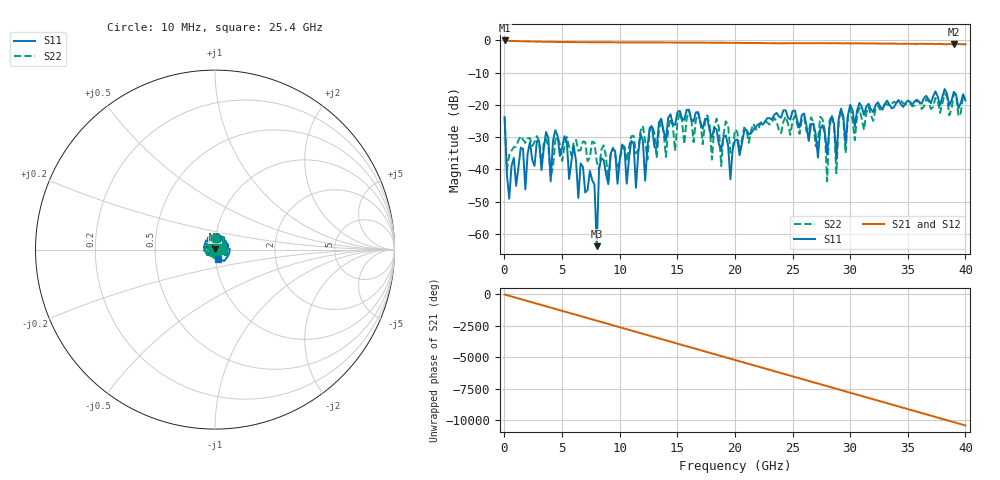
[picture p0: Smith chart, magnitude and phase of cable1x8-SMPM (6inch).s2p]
!Keysight Technologies,N5225A,MY51451228,A.10.40.14
!Date: Monday, November 23, 2020 09:36:10
!Correction: S22(Full 2 Port(2,4))
!S42(Full 2 Port(2,4))
!S24(Full 2 Port(2,4))
!S44(Full 2 Port(2,4))
!S2P File: Measurements: S22, S42, S24, S44:
# Hz S  dB  R 50
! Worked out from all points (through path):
!   201 points, 10 MHz to 40 GHz, reference 50 ohm
!   highest |S21| = -0.01 dB at 10 MHz (marker M1); lowest = -1.2 dB at 39 GHz (marker M2)
!   lowest |S11| = -63.8 dB at 8.008 GHz (marker M3), VSWR 1.00, Z = 50 + j0.0636 ohm
!   |S11| at or under -10 dB: start of sweep to end of sweep
!   |S22| runs from -43.7 to -16.3 dB; largest |S21 - S12| = 0.012
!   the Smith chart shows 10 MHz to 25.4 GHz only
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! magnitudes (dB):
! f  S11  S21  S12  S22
! 10 MHz  -23.8  0.0  -0.1  -24.0
! 409.9 MHz  -49.1  -0.1  -0.1  -35.6
! 3.609 GHz  -28.4  -0.4  -0.4  -30.6
! 4.009 GHz  -43.7  -0.4  -0.4  -42.4
! 4.409 GHz  -27.9  -0.5  -0.5  -30.8
! 6.808 GHz  -39.2  -0.6  -0.5  -31.4
! 7.808 GHz  -44.7  -0.6  -0.6  -31.7
! 8.008 GHz  -63.8  -0.6  -0.5  -37.6
! 8.408 GHz  -36.5  -0.6  -0.6  -33.9
! 11.01 GHz  -31.2  -0.6  -0.6  -29.7
! 11.41 GHz  -45.7  -0.6  -0.6  -35.0
! 13.41 GHz  -25.4  -0.6  -0.6  -27.7
! 20 GHz  -31.0  -0.7  -0.7  -27.6
! 26.8 GHz  -25.8  -0.8  -0.9  -25.3
! 28 GHz  -35.5  -0.9  -0.9  -43.7
! 28.4 GHz  -23.6  -0.9  -0.9  -23.1
! 28.8 GHz  -36.8  -0.9  -0.9  -41.2
! 29.2 GHz  -21.2  -0.9  -0.9  -21.7
! 29.6 GHz  -32.2  -0.9  -0.9  -35.0
! 33.4 GHz  -19.9  -1.0  -1.0  -20.2
! 39 GHz  -15.9  -1.2  -1.2  -16.3
! 40 GHz  -18.6  -1.2  -1.2  -17.5
